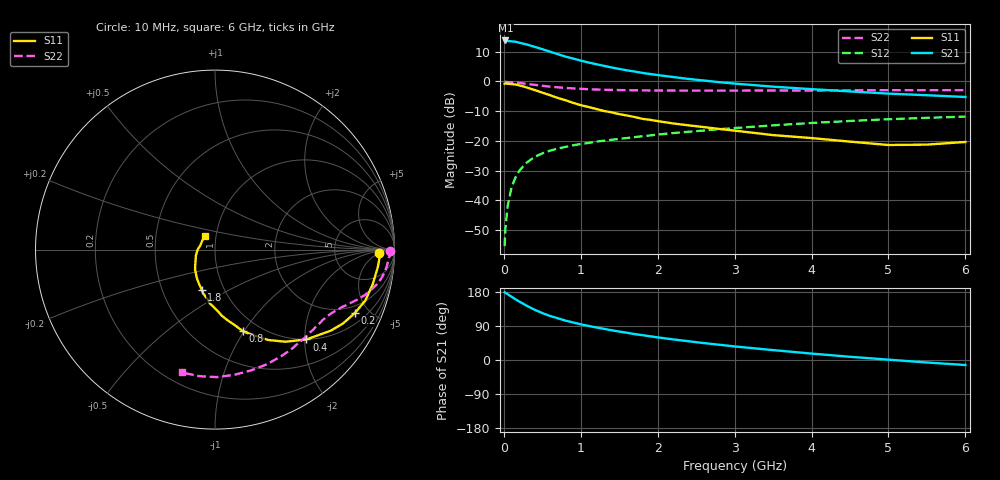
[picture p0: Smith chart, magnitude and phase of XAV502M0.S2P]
! SIEMENS Discrete & RF Semiconductors
! BFY180
! Si NPN RF Bipolar Junction Transistor in MICRO-X
! VCE = 0.5 V  IC = 2 mA
! Common Emitter S-Parameters:  May  1997
# GHz  S  MA  R  50
!  f  S11  S21  S12  S22
! GHz  MAG  ANG  MAG  ANG  MAG  ANG  MAG  ANG
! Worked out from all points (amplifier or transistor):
!   36 points, 10 MHz to 6 GHz, reference 50 ohm
!   highest |S21| = 13.7 dB at 20 MHz (marker M1)
!   |S21| within 3 dB of that: start of sweep to 508.5 MHz
!   unconditionally stable (mu >= 1): 819.9 MHz to end of sweep
!   at 250 MHz: K = 0.36, MSG = 20.6 dB, |S12| = -28.6 dB
!   at 1.4 GHz: K = 1.40, MAG = 8.4 dB, |S12| = -19.6 dB
!   at 6 GHz: K = 1.78, MAG = -1.8 dB, |S12| = -11.9 dB
!   S11 on the Smith chart (normalised r, x): 10 MHz: 21, -5; 200 MHz: 1.54, -4.07; 400 MHz: 1.00, -2.04; 800 MHz: 0.84, -0.99; 1.8 GHz: 0.78, -0.37; 6 GHz: 0.88, +0.14
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0.01  0.9143 -1.3  4.751 178.9  0.0017 86.6  0.9725 -0.4
0.02  0.9179 -2.7  4.863 177.2  0.0033 92.8  0.9838 -1.1
0.05  0.9127 -6.0  4.761 173.5  0.0081 86.1  0.97 -2.6
0.1  0.8995 -12.5  4.71 167.0  0.0165 82.0  0.963 -5.2
0.15  0.884 -18.8  4.625 160.4  0.0241 77.2  0.9543 -7.6
0.2  0.8555 -24.4  4.474 154.2  0.0312 73.4  0.9397 -9.9
0.3  0.7874 -35.0  4.157 142.9  0.0434 66.4  0.9047 -13.8
0.4  0.7141 -44.5  3.803 132.7  0.0539 61.0  0.8733 -16.8
0.5  0.6462 -52.6  3.471 123.8  0.0615 56.7  0.8413 -19.3
0.6  0.5854 -59.4  3.152 116.2  0.0684 53.5  0.814 -21.3
0.8  0.4819 -71.0  2.607 104.0  0.079 49.1  0.7745 -24.5
1  0.3976 -80.2  2.234 94.1  0.0884 46.2  0.7483 -27.5
1.1  0.3706 -84.1  2.071 90.0  0.0923 45.4  0.7375 -28.9
1.4  0.3011 -95.5  1.711 78.4  0.1042 42.9  0.7165 -33.3
1.8  0.2346 -108.6  1.387 65.6  0.1195 41.1  0.7061 -39.3
2.2  0.1962 -119.7  1.182 54.4  0.1351 38.4  0.7 -45.6
2.8  0.1585 -134.4  0.968 40.3  0.1571 34.7  0.6987 -54.8
3.5  0.1249 -150.3  0.814 26.1  0.1822 29.8  0.7014 -65.6
4.5  0.097 -179.9  0.677 8.5  0.2158 20.9  0.7058 -81.2
5  0.0851 163.3  0.622 0.9  0.2307 16.4  0.7105 -89.2
5.5  0.0865 145.9  0.584 -6.6  0.2437 11.8  0.7107 -97.2
6  0.0958 125.5  0.546 -13.2  0.2555 7.1  0.709 -105.1
